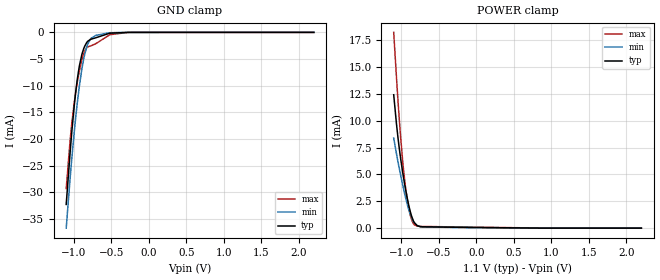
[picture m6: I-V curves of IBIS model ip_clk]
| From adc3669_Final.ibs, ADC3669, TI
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|   ip_clk Model
[Model]   ip_clk
Model_type   Input
Vinl = 0.4
Vinh = 1.3
|   typ   min   max
C_comp   0.3923pF   0.3781pF   0.407pF
| Where C_comp = 0.3923pF at 1.8V, 27C and nominal process
| Where C_comp = 0.407pF at 1.75V, 105C and weak process
| Where C_comp = 0.3781pF at 2V, -40C and strong process
[Voltage Range]   1.8   1.75   2
|Junction Temperature
[Temperature Range]   27   105   -40
[Power Clamp Reference]   1.1   1.05   1.2
[GND Clamp Reference]   0   0   0
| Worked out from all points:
|   GND clamp passes 1 mA (typ) near -0.70 V on its own axis
|   POWER clamp passes 1 mA (typ) near -0.86 V on its own axis
[GND Clamp]
|   Voltage   I(typ)   I(min)   I(max)
-1.1V     -32.3mA    -36.75mA   -29.31mA
-1.047V   -22.4mA    -27.28mA   -20.16mA
-1.024V   -18.49mA   -23.47mA   -16.89mA
-991.1mV  -13.51mA   -18.45mA   -13.01mA
-951.5mV  -8.727mA   -13.16mA   -9.315mA
-925.1mV  -6.341mA   -10.13mA   -7.272mA
-862.4mV  -2.897mA   -4.693mA   -3.819mA
-812.9mV  -1.673mA   -2.209mA   -2.726mA
-766.7mV  -1.268mA   -1.1mA     -2.51mA
-515.9mV  -152.6uA   -62.81uA   -432.4uA
-275mV    -4.274uA   -3.781uA   -8.052uA
2.2V      0A         0A         0A
[POWER Clamp]
|   Voltage   I(typ)   I(min)   I(max)
-1.1V     12.42mA    8.386mA    18.23mA
-1.064V   9.747mA    6.948mA    14.09mA
-1.031V   7.706mA    5.733mA    10.63mA
-1.008V   6.477mA    4.926mA    8.462mA
-974.6mV  4.941mA    3.837mA    5.823mA
-941.6mV  3.597mA    2.836mA    3.77mA
-902mV    2.212mA    1.79mA     1.96mA
-865.7mV  1.212mA    1.037mA    862.3uA
-826.1mV  518.7uA    499.7uA    316.8uA
-786.5mV  226.6uA    235.6uA    186.4uA
-727.1mV  127.3uA    113.3uA    158uA
2.2V      0A         0A         0A
